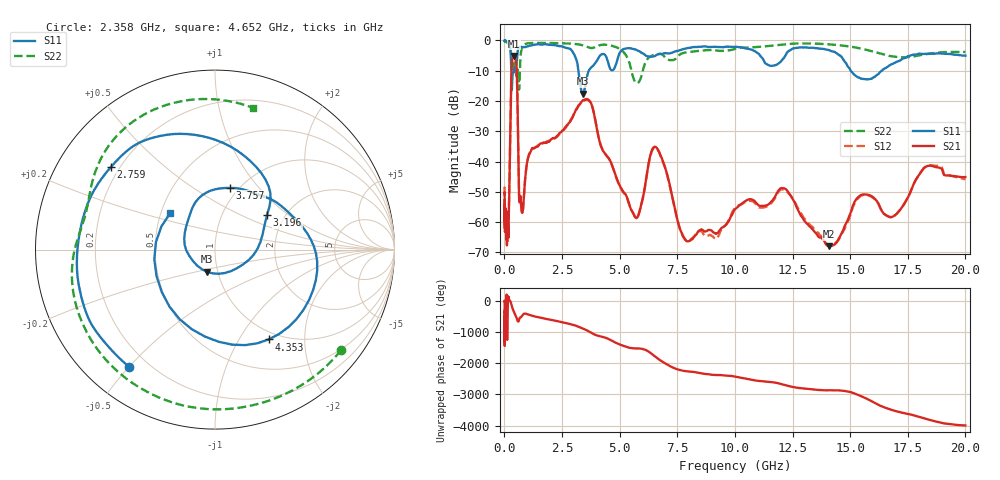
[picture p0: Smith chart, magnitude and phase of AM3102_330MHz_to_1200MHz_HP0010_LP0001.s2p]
! Date/Time: Tue, Sep 11, 2018 5:10 PM
! Network Analyzer: Agilent Technologies E8362B Rev: A.07.50.63
! Sweep from 0.010 to 20.000 GHz, 1601 Points, Sweep Type: LOG
! Power Supply: 4.949 V, 0.001 A
# Hz S DB R 50
!freq MagS11 AngS11 MagS21 AngS21 MagS12 AngS12 MagS22 AngS22
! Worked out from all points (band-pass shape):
!   1601 points, 10 MHz to 20 GHz, reference 50 ohm
!   highest |S21| = -5.16 dB at 406.7 MHz (marker M1); lowest = -67.9 dB at 14.07 GHz (marker M2)
!   |S21| within 3 dB of the highest: 319.6 MHz to 521.9 MHz (202.3 MHz wide, 48.1 % of centre)
!   lowest |S11| = -17.6 dB at 3.4 GHz (marker M3), VSWR 1.30, Z = 44.4 - j11.2 ohm
!   |S11| at or under -10 dB: 297.9 MHz to 358.6 MHz (60.71 MHz wide, 18.5 % of centre); 3.208 GHz to 3.66 GHz (451.9 MHz wide, 13.2 % of centre); 15.03 GHz to 16.37 GHz (1.347 GHz wide, 8.58 % of centre)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
!   |S22| runs from -16.2 to -0.2 dB; largest |S21 - S12| = 0.011
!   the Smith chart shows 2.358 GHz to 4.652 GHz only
!   S11 on the Smith chart (normalised r, x): 2.358 GHz: 0.13, -0.50; 2.759 GHz: 0.17, +0.34; 3.196 GHz: 1.62, +0.70; 3.757 GHz: 0.91, +0.72; 4.353 GHz: 0.89, -1.35; 4.652 GHz: 0.56, +0.26
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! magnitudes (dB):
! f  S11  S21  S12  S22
! 10 MHz  0.0  -50.3  -48.7  -0.2
! 35.55 MHz  0.0  -60.0  -60.6  -0.4
! 126.4 MHz  -0.4  -63.6  -65.2  -0.8
! 181.4 MHz  -1.0  -62.9  -61.3  -1.2
! 308.7 MHz  -14.5  -10.2  -10.2  -6.9
! 406.7 MHz  -10.6  -5.2  -5.2  -8.1
! 447.2 MHz  -9.1  -5.6  -5.6  -7.3
! 757.7 MHz  -2.2  -56.6  -56.8  -2.6
! 1.59 GHz  -1.4  -34.0  -34.1  -0.8
! 2.358 GHz  -1.8  -30.9  -31.2  -0.9
! 2.759 GHz  -2.6  -27.7  -27.8  -1.0
! 3.196 GHz  -9.2  -21.7  -21.9  -1.3
! 3.4 GHz  -17.6  -19.8  -20.0  -1.6
! 3.757 GHz  -9.0  -20.7  -20.7  -2.5
! 4.353 GHz  -4.7  -37.2  -37.2  -1.4
! 4.652 GHz  -9.8  -40.8  -40.9  -1.8
! 5.652 GHz  -2.9  -58.1  -58.1  -13.5
! 6.58 GHz  -4.9  -35.3  -35.5  -4.6
! 7.92 GHz  -2.6  -66.3  -66.2  -3.9
! 12.09 GHz  -6.1  -48.8  -49.1  -1.3
! 14.07 GHz  -3.2  -67.9  -67.5  -1.3
! 20 GHz  -5.0  -45.1  -45.8  -3.8
